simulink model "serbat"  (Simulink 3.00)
settings: Solver=ode45  StartTime=0.0  StopTime=20  MaxStep=0.01  RelTol=1e-5  AbsTol=1e-5
undefined symbols (not defined in the file or in its folder): alfa, hiniz, S, ubar

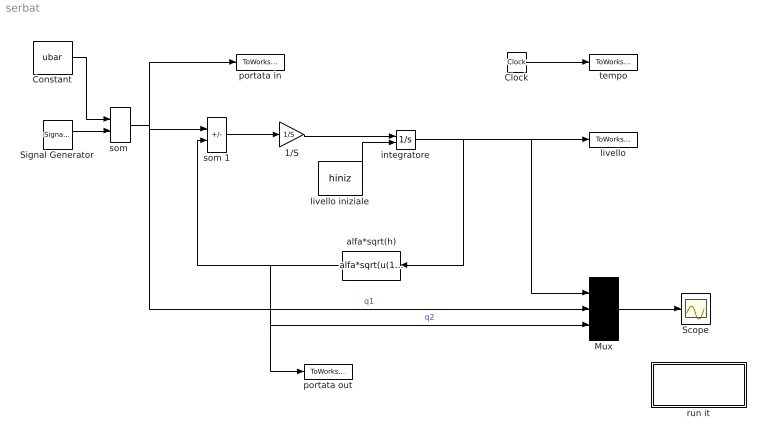
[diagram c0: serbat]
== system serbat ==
  1/S : Gain  Gain=1/S  SaturateOnIntegerOverflow=on
  Clock : Clock
  Constant : Constant  Value=ubar
  Mux : Mux  Inputs=3
  Scope : Scope
  Signal Generator : SignalGenerator  WaveForm=sine  Amplitude=0.5  Frequency=0.2  Units=Hertz
  alfa*sqrt(h) : Fcn  Orientation=left  Expr=alfa*sqrt(u(1))
  integratore : Integrator  ExternalReset=none  InitialConditionSource=external  InitialCondition=hiniz  LimitOutput=off  UpperSaturationLimit=inf  LowerSaturationLimit=-inf  ShowSaturationPort=off  ShowStatePort=off  AbsoluteTolerance=auto
  livello : ToWorkspace  VariableName=h  SampleTime=0  SaveFormat=Matrix
  livello iniziale : Constant  Value=hiniz
  portata in : ToWorkspace  VariableName=q1  SampleTime=0  SaveFormat=Matrix
  portata out : ToWorkspace  VariableName=q2  SampleTime=0  SaveFormat=Matrix
  run it : Subsystem  Description=plot
  "som " : Sum  Inputs=++  SaturateOnIntegerOverflow=on
  som 1 : Sum  Inputs=+-  SaturateOnIntegerOverflow=on
  tempo : ToWorkspace  VariableName=t  SampleTime=0  SaveFormat=Matrix
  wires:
  Clock/1 -> tempo/1
  Constant/1 -> "som "/1
  Signal Generator/1 -> "som "/2
  som 1/1 -> 1/S/1
  "som "/1 -> som 1/1, Mux/2, portata in/1  "q1"
  livello iniziale/1 -> integratore/2
  1/S/1 -> integratore/1
  integratore/1 -> Mux/1, livello/1, alfa*sqrt(h)/1
  Mux/1 -> Scope/1
  alfa*sqrt(h)/1 -> som 1/2, Mux/3, portata out/1  "q2"

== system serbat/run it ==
